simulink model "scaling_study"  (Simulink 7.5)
settings: Solver=ode23t  StartTime=0.0  StopTime=6  RelTol=1e-6
undefined symbols (not defined in the file or in its folder): dfilt, DiscIntNeverNeededParam
libraries: powerlib x45, powerlib_extras x17, simulink x12, dsparch4 x2
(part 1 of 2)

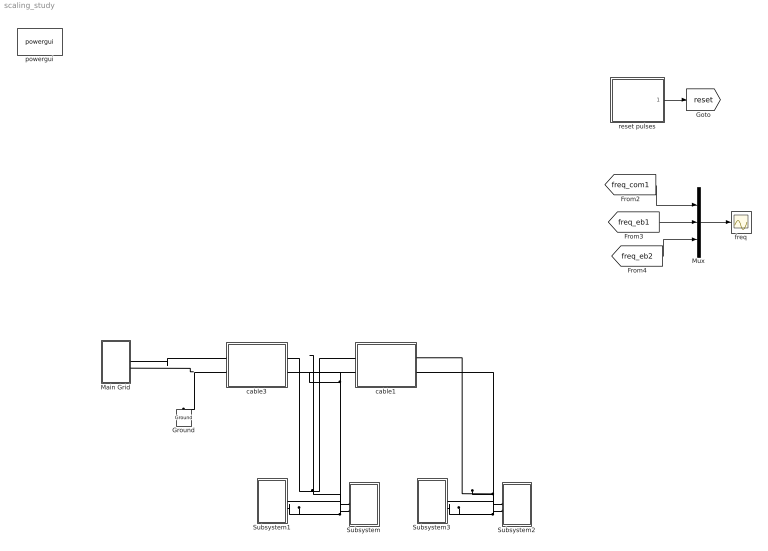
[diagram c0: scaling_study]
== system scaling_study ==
  Ground : powerlib/Elements/Ground  DialogController=POWERSYS.PowerSysDialog  PhysicalDomain=powersysdomain  SubClassName=unknown  LeftPortType=p1  RightPortType=p1  LConnTagsString=a
  Main Grid : Subsystem
  Mux : Mux  Inputs=3
  Subsystem : Subsystem
  Subsystem1 : Subsystem
  Subsystem2 : Subsystem
  Subsystem3 : Subsystem
  cable1 : Subsystem
  cable3 : Subsystem
  freq : Scope
  powergui : powerlib/powergui  Priority=1  SystemSampleTime=-1  SimulationMode=Discrete  SampleTime=50e-5  frequency=60  SPID=off  DisableSnubberDevices=off  DisableRonSwitches=off  DisableVfSwitches=off  SwTol=0  Interpol=off  frequencyindice=0  echomessages=off  HookPort=off  DisplayEquations=off  FunctionMessages=off  EnableUseOfTLC=off  x0status=blocks  RestoreLinks=warning  ResistiveCurrentMeasurement=off  Frange=[0:2:500]  Ylog=off  Xlog=on  ShowGrid=off  save=off  variable=ZData  ZoomFFT=on  StartTime=0.0  cycles=1  DisplayStyle=1  fundamental=60  FreqAxis=off  MaxFrequency=1000  frequencyindicesteady=1  RmsSteady=1  display=off  Ts=0  methode=off
  reset pulses : Subsystem  mask{tpulse=[50 100]}
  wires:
  Mux/1 -> freq/1
  reset pulses/1(Out1) -> [reset]
  [freq_com1] -> Mux/1
  [freq_eb1] -> Mux/2
  [freq_eb2] -> Mux/3
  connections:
  Main Grid/LConn1 -- cable3/RConn1
  cable3/RConn2 -- Main Grid/LConn2 -- Ground/LConn1
  Subsystem/LConn1 -- cable3/LConn1 -- cable1/RConn1 -- Subsystem1/LConn1
  Subsystem/LConn2 -- cable3/LConn2 -- cable1/RConn2 -- Subsystem1/LConn2
  Subsystem2/LConn1 -- cable1/LConn1 -- Subsystem3/LConn1
  Subsystem2/LConn2 -- cable1/LConn2 -- Subsystem3/LConn2

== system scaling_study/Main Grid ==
  " main-grid" : Scope  NumInputPorts=4
  Breaker : powerlib/Elements/Breaker  DialogController=POWERSYS.PowerSysDialog  SystemSampleTime=-1  BreakerResistance=0.01  InitialState=1  SnubberResistance=1e6  SnubberCapacitance=inf  SwitchingTimes=[5]  External=off  Measurements=None  MoreParameters=off  NoBreakLoop=off
  Main Grid 240V rms : powerlib/Electrical Sources/AC Voltage Source  DialogController=POWERSYS.PowerSysDialog  SystemSampleTime=-1  Amplitude=240*sqrt(2)  Phase=0  Frequency=60  SampleTime=0  Measurements=None
  cable : Subsystem
  measurement feeder C5 : Subsystem
  Conn1 : PMIOPort  Port=1  Side=Left
  Conn2 : PMIOPort  Port=2  Side=Left
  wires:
  measurement feeder C5/1(Vm) -> " main-grid"/1
  measurement feeder C5/2(Im) -> " main-grid"/2
  measurement feeder C5/3(PQ) -> " main-grid"/3
  measurement feeder C5/4(RMS (V-I)) -> " main-grid"/4
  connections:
  measurement feeder C5/RConn1 -- Breaker/LConn1
  cable/RConn1 -- Breaker/RConn1
  measurement feeder C5/LConn2 -- Main Grid 240V rms/LConn1
  measurement feeder C5/LConn1 -- Main Grid 240V rms/RConn1
  cable/RConn2 -- measurement feeder C5/RConn2
  Conn1/RConn1 -- cable/LConn1
  Conn2/RConn1 -- cable/LConn2

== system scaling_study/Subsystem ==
  120 Watt  e-board3 : Subsystem  mask{tf=100, p=1}
      mask prompts: tf "fault_time"; p "load priority"
  Breaker2 : powerlib/Elements/Breaker  DialogController=POWERSYS.PowerSysDialog  SystemSampleTime=-1  BreakerResistance=0.01  InitialState=1  SnubberResistance=1e6  SnubberCapacitance=inf  SwitchingTimes=[100]  External=off  Measurements=None  MoreParameters=off  NoBreakLoop=off
  eboard3 : Scope  NumInputPorts=4
  A : PMIOPort  Port=1  Side=Left
  C : PMIOPort  Port=2  Side=Left
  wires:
  120 Watt  e-board3/1(w) -> eboard3/1
  120 Watt  e-board3/2(Irms) -> eboard3/2
  120 Watt  e-board3/3(Vrms) -> eboard3/3
  [reset] -> 120 Watt  e-board3/1(reset)
  120 Watt  e-board3/4(Pload) -> eboard3/4, [Pload3]
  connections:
  120 Watt  e-board3/LConn1 -- Breaker2/LConn1
  A/RConn1 -- Breaker2/RConn1
  C/RConn1 -- 120 Watt  e-board3/LConn2

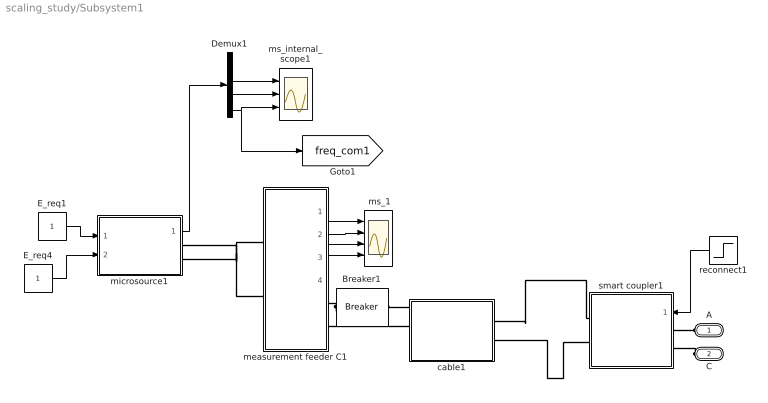
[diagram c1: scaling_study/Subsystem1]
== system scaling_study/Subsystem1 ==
  " ms_1" : Scope  NumInputPorts=4
  Breaker1 : powerlib/Elements/Breaker  DialogController=POWERSYS.PowerSysDialog  SystemSampleTime=-1  BreakerResistance=0.01  InitialState=1  SnubberResistance=1e6  SnubberCapacitance=inf  SwitchingTimes=[100]  External=off  Measurements=None  MoreParameters=off  NoBreakLoop=off
  Demux1 : Demux  Outputs=3
  E_req1 : Constant  OutDataType=fixdt(1, 16)  OutScaling=2^0
  E_req4 : Constant  OutDataType=fixdt(1, 16)  OutScaling=2^0
  cable1 : Subsystem
  measurement feeder C1 : Subsystem
  microsource1 : Subsystem  AncestorBlock=|
      | UWM_blocks/inverter-based
      | DG (simplified)
      | 208V - 15kVA
  ms_internal_scope1 : Scope  NumInputPorts=3
  reconnect1 : Step  Time=.1  SampleTime=0
  smart coupler1 : Subsystem
  A : PMIOPort  Port=1  Side=Left
  C : PMIOPort  Port=2  Side=Left
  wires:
  measurement feeder C1/1(Vm) -> " ms_1"/1
  measurement feeder C1/2(Im) -> " ms_1"/2
  measurement feeder C1/3(PQ) -> " ms_1"/3
  measurement feeder C1/4(RMS (V-I)) -> " ms_1"/4
  E_req1/1 -> microsource1/1(E_req)
  Demux1/2 -> ms_internal_scope1/2
  Demux1/1 -> ms_internal_scope1/1
  Demux1/3 -> ms_internal_scope1/3, [freq_com1]
  microsource1/1(m) -> Demux1/1
  reconnect1/1 -> smart coupler1/1(switch)
  E_req4/1 -> microsource1/2(P_req)
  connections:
  cable1/RConn1 -- Breaker1/LConn1
  Breaker1/RConn1 -- measurement feeder C1/RConn1
  smart coupler1/RConn1 -- cable1/LConn1
  cable1/LConn2 -- smart coupler1/RConn2
  cable1/RConn2 -- measurement feeder C1/RConn2
  measurement feeder C1/LConn1 -- microsource1/RConn1
  measurement feeder C1/LConn2 -- microsource1/RConn2
  A/RConn1 -- smart coupler1/LConn1
  C/RConn1 -- smart coupler1/LConn2

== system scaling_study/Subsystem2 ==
  120 Watt  e-board3 : Subsystem  mask{tf=100, p=1}
      mask prompts: tf "fault_time"; p "load priority"
  Breaker2 : powerlib/Elements/Breaker  DialogController=POWERSYS.PowerSysDialog  SystemSampleTime=-1  BreakerResistance=0.01  InitialState=1  SnubberResistance=1e6  SnubberCapacitance=inf  SwitchingTimes=[100]  External=off  Measurements=None  MoreParameters=off  NoBreakLoop=off
  eboard3 : Scope  NumInputPorts=4
  A : PMIOPort  Port=1  Side=Left
  C : PMIOPort  Port=2  Side=Left
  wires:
  120 Watt  e-board3/1(w) -> eboard3/1
  120 Watt  e-board3/2(Irms) -> eboard3/2
  120 Watt  e-board3/3(Vrms) -> eboard3/3
  [reset] -> 120 Watt  e-board3/1(reset)
  120 Watt  e-board3/4(Pload) -> eboard3/4, [Pload3]
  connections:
  120 Watt  e-board3/LConn1 -- Breaker2/LConn1
  A/RConn1 -- Breaker2/RConn1
  C/RConn1 -- 120 Watt  e-board3/LConn2

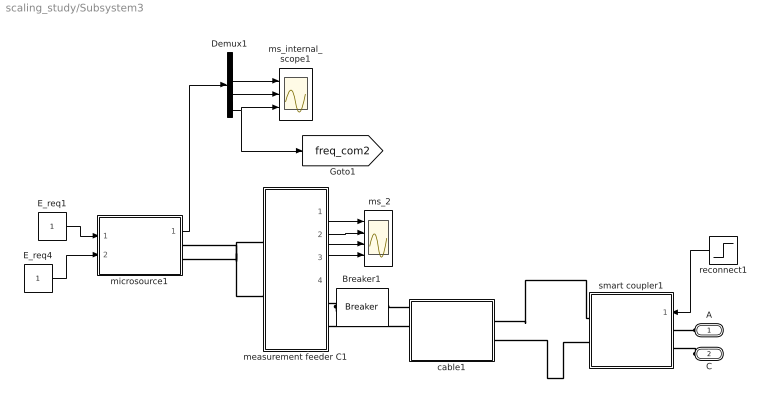
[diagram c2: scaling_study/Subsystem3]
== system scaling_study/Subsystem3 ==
  " ms_2" : Scope  NumInputPorts=4
  Breaker1 : powerlib/Elements/Breaker  DialogController=POWERSYS.PowerSysDialog  SystemSampleTime=-1  BreakerResistance=0.01  InitialState=1  SnubberResistance=1e6  SnubberCapacitance=inf  SwitchingTimes=[100]  External=off  Measurements=None  MoreParameters=off  NoBreakLoop=off
  Demux1 : Demux  Outputs=3
  E_req1 : Constant  OutDataType=fixdt(1, 16)  OutScaling=2^0
  E_req4 : Constant  OutDataType=fixdt(1, 16)  OutScaling=2^0
  cable1 : Subsystem
  measurement feeder C1 : Subsystem
  microsource1 : Subsystem  AncestorBlock=|
      | UWM_blocks/inverter-based
      | DG (simplified)
      | 208V - 15kVA
  ms_internal_scope1 : Scope  NumInputPorts=3
  reconnect1 : Step  Time=.1  SampleTime=0
  smart coupler1 : Subsystem
  A : PMIOPort  Port=1  Side=Left
  C : PMIOPort  Port=2  Side=Left
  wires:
  measurement feeder C1/1(Vm) -> " ms_2"/1
  measurement feeder C1/2(Im) -> " ms_2"/2
  measurement feeder C1/3(PQ) -> " ms_2"/3
  measurement feeder C1/4(RMS (V-I)) -> " ms_2"/4
  E_req1/1 -> microsource1/1(E_req)
  Demux1/2 -> ms_internal_scope1/2
  Demux1/1 -> ms_internal_scope1/1
  Demux1/3 -> ms_internal_scope1/3, [freq_com2]
  microsource1/1(m) -> Demux1/1
  reconnect1/1 -> smart coupler1/1(switch)
  E_req4/1 -> microsource1/2(P_req)
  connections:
  cable1/RConn1 -- Breaker1/LConn1
  Breaker1/RConn1 -- measurement feeder C1/RConn1
  smart coupler1/RConn1 -- cable1/LConn1
  cable1/LConn2 -- smart coupler1/RConn2
  cable1/RConn2 -- measurement feeder C1/RConn2
  measurement feeder C1/LConn1 -- microsource1/RConn1
  measurement feeder C1/LConn2 -- microsource1/RConn2
  A/RConn1 -- smart coupler1/LConn1
  C/RConn1 -- smart coupler1/LConn2

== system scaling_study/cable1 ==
  Series RLC Branch : powerlib/Elements/Series RLC Branch  DialogController=POWERSYS.PowerSysDialog  PhysicalDomain=powersysdomain  SubClassName=unknown  LeftPortType=p1  RightPortType=p1  LConnTagsString=__new0  RConnTagsString=__new0  BranchType=RL  Resistance=.001  Inductance=1.e-6  SetiL0=off  InitialCurrent=0  Capacitance=1e-6  Setx0=off  InitialVoltage=0  Measurements=None
  A : PMIOPort  Tag=PMCPort  Port=1  Side=Left
  A' : PMIOPort  Tag=PMCPort  Port=2  Side=Right
  B' : PMIOPort  Tag=PMCPort  Port=3  Side=Right
  B : PMIOPort  Tag=PMCPort  Port=4  Side=Left
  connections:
  A/RConn1 -- Series RLC Branch/LConn1
  Series RLC Branch/RConn1 -- A'/RConn1
  B/RConn1 -- B'/RConn1

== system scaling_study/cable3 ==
  Series RLC Branch : powerlib/Elements/Series RLC Branch  DialogController=POWERSYS.PowerSysDialog  PhysicalDomain=powersysdomain  SubClassName=unknown  LeftPortType=p1  RightPortType=p1  LConnTagsString=__new0  RConnTagsString=__new0  BranchType=RL  Resistance=.001  Inductance=1.e-6  SetiL0=off  InitialCurrent=0  Capacitance=1e-6  Setx0=off  InitialVoltage=0  Measurements=None
  A : PMIOPort  Tag=PMCPort  Port=1  Side=Left
  A' : PMIOPort  Tag=PMCPort  Port=2  Side=Right
  B' : PMIOPort  Tag=PMCPort  Port=3  Side=Right
  B : PMIOPort  Tag=PMCPort  Port=4  Side=Left
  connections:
  A/RConn1 -- Series RLC Branch/LConn1
  Series RLC Branch/RConn1 -- A'/RConn1
  B/RConn1 -- B'/RConn1

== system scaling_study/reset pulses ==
  Sum : Sum  Inputs=|++  OutDataType=fixdt(1, 16)  OutScaling=2^0
  pulse : Subsystem  mask{tstart=tpulse(1), dt=.1}
  pulse1 : Subsystem  mask{tstart=tpulse(2), dt=.1}
  Out1 : Outport
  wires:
  pulse/1(Out1) -> Sum/1
  pulse1/1(Out1) -> Sum/2
  Sum/1 -> Out1/1

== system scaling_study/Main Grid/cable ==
  Series RLC Branch : powerlib/Elements/Series RLC Branch  DialogController=POWERSYS.PowerSysDialog  PhysicalDomain=powersysdomain  SubClassName=unknown  LeftPortType=p1  RightPortType=p1  LConnTagsString=__new0  RConnTagsString=__new0  BranchType=RL  Resistance=.001  Inductance=1.e-5  SetiL0=off  InitialCurrent=0  Capacitance=1e-6  Setx0=off  InitialVoltage=0  Measurements=None
  A : PMIOPort  Tag=PMCPort  Port=1  Side=Left
  A' : PMIOPort  Tag=PMCPort  Port=2  Side=Right
  B' : PMIOPort  Tag=PMCPort  Port=3  Side=Right
  B : PMIOPort  Tag=PMCPort  Port=4  Side=Left
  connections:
  A/RConn1 -- Series RLC Branch/LConn1
  A'/RConn1 -- Series RLC Branch/RConn1
  B/RConn1 -- B'/RConn1

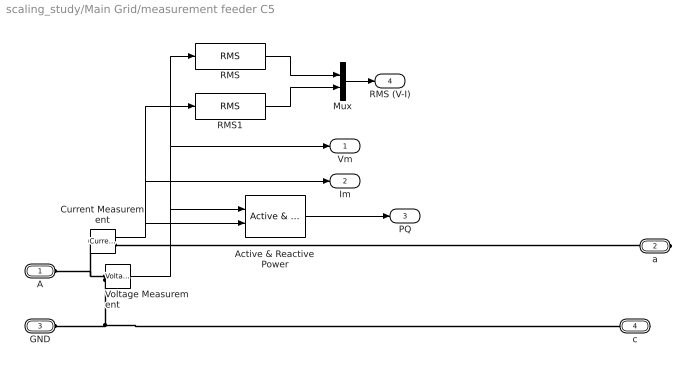
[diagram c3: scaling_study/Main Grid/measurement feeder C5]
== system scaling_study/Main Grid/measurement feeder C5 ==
  Active & Reactive Power : powerlib_extras/Measurements/Active & Reactive Power  DialogController=POWERSYS.PowerSysDialog  SystemSampleTime=-1  f1=60
  Current Measurement : powerlib/Measurements/Current Measurement  DialogController=POWERSYS.PowerSysDialog  SystemSampleTime=-1  PhasorSimulation=off  OutputType=Complex  PSBequivalent=0
  Mux : Mux  Inputs=2
  RMS : powerlib_extras/Measurements/RMS  DialogController=POWERSYS.PowerSysDialog  SystemSampleTime=-1  f1=60
  RMS1 : powerlib_extras/Measurements/RMS  DialogController=POWERSYS.PowerSysDialog  SystemSampleTime=-1  f1=60
  Voltage Measurement : powerlib/Measurements/Voltage Measurement  DialogController=POWERSYS.PowerSysDialog  SystemSampleTime=-1  PhasorSimulation=off  OutputType=Complex  PSBequivalent=0
  A : PMIOPort  Port=1  Side=Left
  a : PMIOPort  Port=2  Side=Right
  GND : PMIOPort  Port=3  Side=Left
  c : PMIOPort  Port=4  Side=Right
  Vm : Outport  OutDataType=fixdt(1, 16)  OutScaling=2^0
  Im : Outport  Port=2  OutDataType=fixdt(1, 16)  OutScaling=2^0
  PQ : Outport  Port=3  OutDataType=fixdt(1, 16)  OutScaling=2^0
  RMS (V-I) : Outport  Port=4  OutDataType=fixdt(1, 16)  OutScaling=2^0
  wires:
  Mux/1 -> RMS (V-I)/1
  Current Measurement/1 -> Im/1, RMS1/1, Active & Reactive Power/2
  Voltage Measurement/1 -> Vm/1, RMS/1, Active & Reactive Power/1
  Active & Reactive Power/1 -> PQ/1
  RMS/1 -> Mux/1
  RMS1/1 -> Mux/2
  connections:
  a/RConn1 -- Current Measurement/RConn1
  Voltage Measurement/LConn1 -- A/RConn1 -- Current Measurement/LConn1
  Voltage Measurement/LConn2 -- GND/RConn1 -- c/RConn1

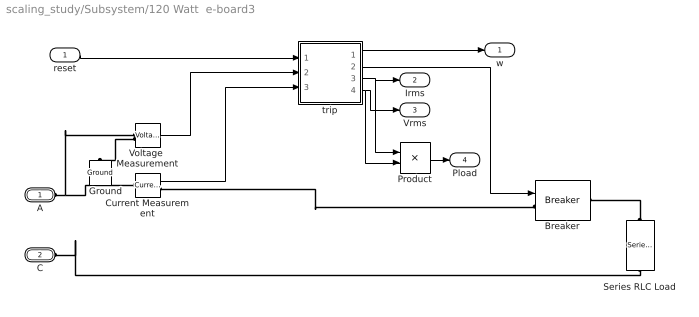
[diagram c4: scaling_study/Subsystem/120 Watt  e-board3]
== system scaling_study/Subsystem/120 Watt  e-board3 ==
  reset : Inport
  Breaker : powerlib/Elements/Breaker  DialogController=POWERSYS.PowerSysDialog  SystemSampleTime=-1  BreakerResistance=0.01  InitialState=1  SnubberResistance=1e6  SnubberCapacitance=inf  SwitchingTimes="[ 1/60  5/60 ]"  External=on  Measurements=None  MoreParameters=off  NoBreakLoop=off
  Current Measurement : powerlib/Measurements/Current Measurement  DialogController=POWERSYS.PowerSysDialog  SystemSampleTime=-1  PhasorSimulation=off  OutputType=Complex  PSBequivalent=0
  Ground : powerlib/Elements/Ground  DialogController=POWERSYS.PowerSysDialog  PhysicalDomain=powersysdomain  SubClassName=unknown  LeftPortType=p1  RightPortType=p1  LConnTagsString=a
  Product : Product  OutDataType=fixdt(1, 16)  OutScaling=2^0
  Series RLC Load : powerlib/Elements/Series RLC Load  DialogController=POWERSYS.PowerSysDialog  PhysicalDomain=powersysdomain  SubClassName=unknown  LeftPortType=p1  RightPortType=p1  LConnTagsString=a  RConnTagsString=__new0  NominalVoltage=240  NominalFrequency=60  ActivePower=120  InductivePower=0  CapacitivePower=0  Setx0=off  InitialVoltage=0  SetiL0=off  InitialCurrent=0  Measurements=None
  Voltage  Measurement : powerlib/Measurements/Voltage Measurement  DialogController=POWERSYS.PowerSysDialog  SystemSampleTime=-1  PhasorSimulation=off  OutputType=Complex  PSBequivalent=0
  trip : Subsystem  mask{p=p}
      mask prompts: p "priority level"
  A : PMIOPort  Port=1  Side=Left
  C : PMIOPort  Port=2  Side=Left
  w : Outport  OutDataType=fixdt(1, 16)  OutScaling=2^0
  Irms : Outport  Port=2  OutDataType=fixdt(1, 16)  OutScaling=2^0
  Vrms : Outport  Port=3  OutDataType=fixdt(1, 16)  OutScaling=2^0
  Pload : Outport  Port=4  OutDataType=fixdt(1, 16)  OutScaling=2^0
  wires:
  trip/1(w) -> w/1
  Current Measurement/1 -> trip/3(I)
  Voltage  Measurement/1 -> trip/2(V)
  reset/1 -> trip/1(Reset)
  trip/2(trip) -> Breaker/1
  trip/3(Irms) -> Irms/1, Product/1
  trip/4(Vrms) -> Vrms/1, Product/2
  Product/1 -> Pload/1
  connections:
  A/RConn1 -- Current Measurement/LConn1 -- Voltage  Measurement/LConn1
  Voltage  Measurement/LConn2 -- Ground/LConn1
  Current Measurement/RConn1 -- Breaker/LConn1
  Series RLC Load/LConn1 -- Breaker/RConn1
  Series RLC Load/RConn1 -- C/RConn1

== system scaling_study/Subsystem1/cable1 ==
  Series RLC Branch : powerlib/Elements/Series RLC Branch  DialogController=POWERSYS.PowerSysDialog  PhysicalDomain=powersysdomain  SubClassName=unknown  LeftPortType=p1  RightPortType=p1  LConnTagsString=__new0  RConnTagsString=__new0  BranchType=RL  Resistance=.001  Inductance=1.e-6  SetiL0=off  InitialCurrent=0  Capacitance=1e-6  Setx0=off  InitialVoltage=0  Measurements=None
  A : PMIOPort  Tag=PMCPort  Port=1  Side=Left
  A' : PMIOPort  Tag=PMCPort  Port=2  Side=Right
  B' : PMIOPort  Tag=PMCPort  Port=3  Side=Right
  B : PMIOPort  Tag=PMCPort  Port=4  Side=Left
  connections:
  A/RConn1 -- Series RLC Branch/LConn1
  Series RLC Branch/RConn1 -- A'/RConn1
  B/RConn1 -- B'/RConn1

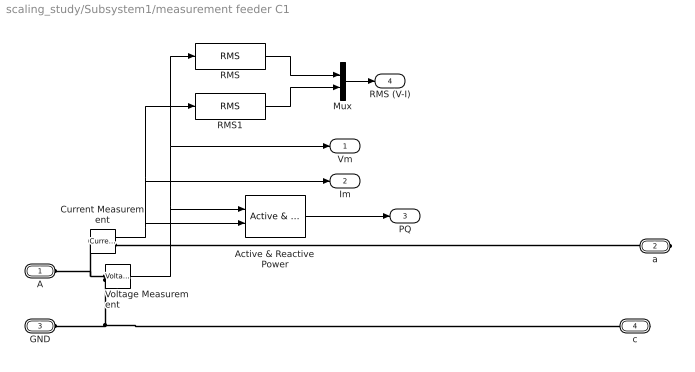
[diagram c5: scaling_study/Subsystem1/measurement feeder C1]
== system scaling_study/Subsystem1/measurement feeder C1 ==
  Active & Reactive Power : powerlib_extras/Measurements/Active & Reactive Power  DialogController=POWERSYS.PowerSysDialog  SystemSampleTime=-1  f1=60
  Current Measurement : powerlib/Measurements/Current Measurement  DialogController=POWERSYS.PowerSysDialog  SystemSampleTime=-1  PhasorSimulation=off  OutputType=Complex  PSBequivalent=0
  Mux : Mux  Inputs=2
  RMS : powerlib_extras/Measurements/RMS  DialogController=POWERSYS.PowerSysDialog  SystemSampleTime=-1  f1=60
  RMS1 : powerlib_extras/Measurements/RMS  DialogController=POWERSYS.PowerSysDialog  SystemSampleTime=-1  f1=60
  Voltage Measurement : powerlib/Measurements/Voltage Measurement  DialogController=POWERSYS.PowerSysDialog  SystemSampleTime=-1  PhasorSimulation=off  OutputType=Complex  PSBequivalent=0
  A : PMIOPort  Port=1  Side=Left
  a : PMIOPort  Port=2  Side=Right
  GND : PMIOPort  Port=3  Side=Left
  c : PMIOPort  Port=4  Side=Right
  Vm : Outport  OutDataType=fixdt(1, 16)  OutScaling=2^0
  Im : Outport  Port=2  OutDataType=fixdt(1, 16)  OutScaling=2^0
  PQ : Outport  Port=3  OutDataType=fixdt(1, 16)  OutScaling=2^0
  RMS (V-I) : Outport  Port=4  OutDataType=fixdt(1, 16)  OutScaling=2^0
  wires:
  Mux/1 -> RMS (V-I)/1
  Current Measurement/1 -> Im/1, RMS1/1, Active & Reactive Power/2
  Voltage Measurement/1 -> Vm/1, RMS/1, Active & Reactive Power/1
  Active & Reactive Power/1 -> PQ/1
  RMS/1 -> Mux/1
  RMS1/1 -> Mux/2
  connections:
  a/RConn1 -- Current Measurement/RConn1
  Voltage Measurement/LConn1 -- A/RConn1 -- Current Measurement/LConn1
  Voltage Measurement/LConn2 -- GND/RConn1 -- c/RConn1

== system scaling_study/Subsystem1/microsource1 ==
  E_req : Inport
  P_req : Inport  Port=2
  Current Measurement : powerlib/Measurements/Current Measurement  DialogController=POWERSYS.PowerSysDialog  SystemSampleTime=-1  PhasorSimulation=off  OutputType=Complex  PSBequivalent=0
  Gain : Gain  Gain=1/(2*pi)  ParameterDataType=fixdt(1, 16)  ParameterScaling=2^0  OutDataType=fixdt(1, 16)  OutScaling=2^0
  Mux : Mux  Inputs=3
  Parallel RLC Branch : powerlib/Elements/Parallel RLC Branch  DialogController=POWERSYS.PowerSysDialog  PhysicalDomain=powersysdomain  SubClassName=unknown  LeftPortType=p1  RightPortType=p1  LConnTagsString=a  RConnTagsString=__new0  BranchType=L  Resistance=1  Inductance=1.e-1  SetiL0=off  InitialCurrent=0  Capacitance=1e-6  Setx0=off  InitialVoltage=0  Measurements=None
  Parallel RLC Branch1 : powerlib/Elements/Parallel RLC Branch  DialogController=POWERSYS.PowerSysDialog  PhysicalDomain=powersysdomain  SubClassName=unknown  LeftPortType=p1  RightPortType=p1  LConnTagsString=a  RConnTagsString=__new0  BranchType=L  Resistance=1  Inductance=1.e-1  SetiL0=off  InitialCurrent=0  Capacitance=1e-6  Setx0=off  InitialVoltage=0  Measurements=None
  Parallel RLC Branch2 : powerlib/Elements/Parallel RLC Branch  DialogController=POWERSYS.PowerSysDialog  PhysicalDomain=powersysdomain  SubClassName=unknown  LeftPortType=p1  RightPortType=p1  LConnTagsString=a  RConnTagsString=__new0  BranchType=C  Resistance=1  Inductance=1.e-1  SetiL0=off  InitialCurrent=0  Capacitance=1.e-5  Setx0=off  InitialVoltage=0  Measurements=None
  UWM_controller : Subsystem  mask{Vbase=240*sqrt(2), Sbase=200}
  Voltage Measurement : powerlib/Measurements/Voltage Measurement  DialogController=POWERSYS.PowerSysDialog  SystemSampleTime=-1  PhasorSimulation=off  OutputType=Complex  PSBequivalent=0
  microsource : Subsystem
  a : PMIOPort  Port=1  Side=Right
  GND : PMIOPort  Port=2  Side=Right
  m : Outport  OutDataType=fixdt(1, 16)  OutScaling=2^0
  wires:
  E_req/1 -> UWM_controller/3(E_req)
  P_req/1 -> UWM_controller/4(P_req)
  UWM_controller/1(Vpk) -> microsource/1(Vpk)
  UWM_controller/2(w) -> microsource/2(w), Gain/1
  Mux/1 -> m/1
  Gain/1 -> Mux/3
  Current Measurement/1 -> Mux/2, UWM_controller/2(i_meas)
  Voltage Measurement/1 -> Mux/1, UWM_controller/1(v_meas)
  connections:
  Voltage Measurement/LConn2 -- GND/RConn1 -- Parallel RLC Branch2/RConn1 -- microsource/RConn2
  Parallel RLC Branch1/RConn1 -- Voltage Measurement/LConn1 -- Current Measurement/LConn1
  a/RConn1 -- Current Measurement/RConn1
  Parallel RLC Branch/LConn1 -- microsource/RConn1
  Parallel RLC Branch2/LConn1 -- Parallel RLC Branch1/LConn1 -- Parallel RLC Branch/RConn1

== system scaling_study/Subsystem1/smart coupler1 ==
  switch : Inport  OutDataType=fixdt(1, 16)  OutScaling=2^0
  Abs : Abs  OutDataType=fixdt(1, 16)  OutScaling=2^0
  Breaker : powerlib/Elements/Breaker  DialogController=POWERSYS.PowerSysDialog  SystemSampleTime=-1  BreakerResistance=0.01  InitialState=0  SnubberResistance=1e6  SnubberCapacitance=inf  SwitchingTimes="[ 1/60  5/60 ]"  External=on  Measurements=None  MoreParameters=off  NoBreakLoop=off
  Level-2 M-file S-Function : M-S-Function  FunctionName=smart_coupler
  Scope : Scope  NumInputPorts=3
  Transfer Fcn : TransferFcn  Numerator=[100]  Denominator=[1 100]
  Voltage Measurement : powerlib/Measurements/Voltage Measurement  DialogController=POWERSYS.PowerSysDialog  SystemSampleTime=-1  PhasorSimulation=off  OutputType=Complex  PSBequivalent=0
  A : PMIOPort  Port=1  Side=Left
  C : PMIOPort  Port=2  Side=Left
  a : PMIOPort  Port=3  Side=Right
  c : PMIOPort  Port=4  Side=Right
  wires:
  switch/1 -> Level-2 M-file S-Function/2, Scope/2
  Level-2 M-file S-Function/1 -> Scope/1, Breaker/1
  Voltage Measurement/1 -> Abs/1
  Abs/1 -> Transfer Fcn/1
  Transfer Fcn/1 -> Level-2 M-file S-Function/1, Scope/3
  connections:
  Breaker/LConn1 -- A/RConn1 -- Voltage Measurement/LConn1
  Breaker/RConn1 -- Voltage Measurement/LConn2 -- a/RConn1
  c/RConn1 -- C/RConn1

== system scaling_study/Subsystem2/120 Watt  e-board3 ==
  reset : Inport
  Breaker : powerlib/Elements/Breaker  DialogController=POWERSYS.PowerSysDialog  SystemSampleTime=-1  BreakerResistance=0.01  InitialState=1  SnubberResistance=1e6  SnubberCapacitance=inf  SwitchingTimes="[ 1/60  5/60 ]"  External=on  Measurements=None  MoreParameters=off  NoBreakLoop=off
  Current Measurement : powerlib/Measurements/Current Measurement  DialogController=POWERSYS.PowerSysDialog  SystemSampleTime=-1  PhasorSimulation=off  OutputType=Complex  PSBequivalent=0
  Ground : powerlib/Elements/Ground  DialogController=POWERSYS.PowerSysDialog  PhysicalDomain=powersysdomain  SubClassName=unknown  LeftPortType=p1  RightPortType=p1  LConnTagsString=a
  Product : Product  OutDataType=fixdt(1, 16)  OutScaling=2^0
  Series RLC Load : powerlib/Elements/Series RLC Load  DialogController=POWERSYS.PowerSysDialog  PhysicalDomain=powersysdomain  SubClassName=unknown  LeftPortType=p1  RightPortType=p1  LConnTagsString=a  RConnTagsString=__new0  NominalVoltage=240  NominalFrequency=60  ActivePower=120  InductivePower=0  CapacitivePower=0  Setx0=off  InitialVoltage=0  SetiL0=off  InitialCurrent=0  Measurements=None
  Voltage  Measurement : powerlib/Measurements/Voltage Measurement  DialogController=POWERSYS.PowerSysDialog  SystemSampleTime=-1  PhasorSimulation=off  OutputType=Complex  PSBequivalent=0
  trip : Subsystem  mask{p=p}
      mask prompts: p "priority level"
  A : PMIOPort  Port=1  Side=Left
  C : PMIOPort  Port=2  Side=Left
  w : Outport  OutDataType=fixdt(1, 16)  OutScaling=2^0
  Irms : Outport  Port=2  OutDataType=fixdt(1, 16)  OutScaling=2^0
  Vrms : Outport  Port=3  OutDataType=fixdt(1, 16)  OutScaling=2^0
  Pload : Outport  Port=4  OutDataType=fixdt(1, 16)  OutScaling=2^0
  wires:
  trip/1(w) -> w/1
  Current Measurement/1 -> trip/3(I)
  Voltage  Measurement/1 -> trip/2(V)
  reset/1 -> trip/1(Reset)
  trip/2(trip) -> Breaker/1
  trip/3(Irms) -> Irms/1, Product/1
  trip/4(Vrms) -> Vrms/1, Product/2
  Product/1 -> Pload/1
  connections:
  A/RConn1 -- Current Measurement/LConn1 -- Voltage  Measurement/LConn1
  Voltage  Measurement/LConn2 -- Ground/LConn1
  Current Measurement/RConn1 -- Breaker/LConn1
  Series RLC Load/LConn1 -- Breaker/RConn1
  Series RLC Load/RConn1 -- C/RConn1

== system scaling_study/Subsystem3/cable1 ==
  Series RLC Branch : powerlib/Elements/Series RLC Branch  DialogController=POWERSYS.PowerSysDialog  PhysicalDomain=powersysdomain  SubClassName=unknown  LeftPortType=p1  RightPortType=p1  LConnTagsString=__new0  RConnTagsString=__new0  BranchType=RL  Resistance=.001  Inductance=1.e-6  SetiL0=off  InitialCurrent=0  Capacitance=1e-6  Setx0=off  InitialVoltage=0  Measurements=None
  A : PMIOPort  Tag=PMCPort  Port=1  Side=Left
  A' : PMIOPort  Tag=PMCPort  Port=2  Side=Right
  B' : PMIOPort  Tag=PMCPort  Port=3  Side=Right
  B : PMIOPort  Tag=PMCPort  Port=4  Side=Left
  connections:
  A/RConn1 -- Series RLC Branch/LConn1
  Series RLC Branch/RConn1 -- A'/RConn1
  B/RConn1 -- B'/RConn1

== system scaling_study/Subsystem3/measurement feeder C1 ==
  Active & Reactive Power : powerlib_extras/Measurements/Active & Reactive Power  DialogController=POWERSYS.PowerSysDialog  SystemSampleTime=-1  f1=60
  Current Measurement : powerlib/Measurements/Current Measurement  DialogController=POWERSYS.PowerSysDialog  SystemSampleTime=-1  PhasorSimulation=off  OutputType=Complex  PSBequivalent=0
  Mux : Mux  Inputs=2
  RMS : powerlib_extras/Measurements/RMS  DialogController=POWERSYS.PowerSysDialog  SystemSampleTime=-1  f1=60
  RMS1 : powerlib_extras/Measurements/RMS  DialogController=POWERSYS.PowerSysDialog  SystemSampleTime=-1  f1=60
  Voltage Measurement : powerlib/Measurements/Voltage Measurement  DialogController=POWERSYS.PowerSysDialog  SystemSampleTime=-1  PhasorSimulation=off  OutputType=Complex  PSBequivalent=0
  A : PMIOPort  Port=1  Side=Left
  a : PMIOPort  Port=2  Side=Right
  GND : PMIOPort  Port=3  Side=Left
  c : PMIOPort  Port=4  Side=Right
  Vm : Outport  OutDataType=fixdt(1, 16)  OutScaling=2^0
  Im : Outport  Port=2  OutDataType=fixdt(1, 16)  OutScaling=2^0
  PQ : Outport  Port=3  OutDataType=fixdt(1, 16)  OutScaling=2^0
  RMS (V-I) : Outport  Port=4  OutDataType=fixdt(1, 16)  OutScaling=2^0
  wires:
  Mux/1 -> RMS (V-I)/1
  Current Measurement/1 -> Im/1, RMS1/1, Active & Reactive Power/2
  Voltage Measurement/1 -> Vm/1, RMS/1, Active & Reactive Power/1
  Active & Reactive Power/1 -> PQ/1
  RMS/1 -> Mux/1
  RMS1/1 -> Mux/2
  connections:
  a/RConn1 -- Current Measurement/RConn1
  Voltage Measurement/LConn1 -- A/RConn1 -- Current Measurement/LConn1
  Voltage Measurement/LConn2 -- GND/RConn1 -- c/RConn1

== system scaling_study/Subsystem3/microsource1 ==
  E_req : Inport
  P_req : Inport  Port=2
  Current Measurement : powerlib/Measurements/Current Measurement  DialogController=POWERSYS.PowerSysDialog  SystemSampleTime=-1  PhasorSimulation=off  OutputType=Complex  PSBequivalent=0
  Gain : Gain  Gain=1/(2*pi)  ParameterDataType=fixdt(1, 16)  ParameterScaling=2^0  OutDataType=fixdt(1, 16)  OutScaling=2^0
  Mux : Mux  Inputs=3
  Parallel RLC Branch : powerlib/Elements/Parallel RLC Branch  DialogController=POWERSYS.PowerSysDialog  PhysicalDomain=powersysdomain  SubClassName=unknown  LeftPortType=p1  RightPortType=p1  LConnTagsString=a  RConnTagsString=__new0  BranchType=L  Resistance=1  Inductance=1.e-1  SetiL0=off  InitialCurrent=0  Capacitance=1e-6  Setx0=off  InitialVoltage=0  Measurements=None
  Parallel RLC Branch1 : powerlib/Elements/Parallel RLC Branch  DialogController=POWERSYS.PowerSysDialog  PhysicalDomain=powersysdomain  SubClassName=unknown  LeftPortType=p1  RightPortType=p1  LConnTagsString=a  RConnTagsString=__new0  BranchType=L  Resistance=1  Inductance=1.e-1  SetiL0=off  InitialCurrent=0  Capacitance=1e-6  Setx0=off  InitialVoltage=0  Measurements=None
  Parallel RLC Branch2 : powerlib/Elements/Parallel RLC Branch  DialogController=POWERSYS.PowerSysDialog  PhysicalDomain=powersysdomain  SubClassName=unknown  LeftPortType=p1  RightPortType=p1  LConnTagsString=a  RConnTagsString=__new0  BranchType=C  Resistance=1  Inductance=1.e-1  SetiL0=off  InitialCurrent=0  Capacitance=1.e-5  Setx0=off  InitialVoltage=0  Measurements=None
  UWM_controller : Subsystem  mask{Vbase=240*sqrt(2), Sbase=200}
  Voltage Measurement : powerlib/Measurements/Voltage Measurement  DialogController=POWERSYS.PowerSysDialog  SystemSampleTime=-1  PhasorSimulation=off  OutputType=Complex  PSBequivalent=0
  microsource : Subsystem
  a : PMIOPort  Port=1  Side=Right
  GND : PMIOPort  Port=2  Side=Right
  m : Outport  OutDataType=fixdt(1, 16)  OutScaling=2^0
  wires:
  E_req/1 -> UWM_controller/3(E_req)
  P_req/1 -> UWM_controller/4(P_req)
  UWM_controller/1(Vpk) -> microsource/1(Vpk)
  UWM_controller/2(w) -> microsource/2(w), Gain/1
  Mux/1 -> m/1
  Gain/1 -> Mux/3
  Current Measurement/1 -> Mux/2, UWM_controller/2(i_meas)
  Voltage Measurement/1 -> Mux/1, UWM_controller/1(v_meas)
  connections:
  Voltage Measurement/LConn2 -- GND/RConn1 -- Parallel RLC Branch2/RConn1 -- microsource/RConn2
  Parallel RLC Branch1/RConn1 -- Voltage Measurement/LConn1 -- Current Measurement/LConn1
  a/RConn1 -- Current Measurement/RConn1
  Parallel RLC Branch/LConn1 -- microsource/RConn1
  Parallel RLC Branch2/LConn1 -- Parallel RLC Branch1/LConn1 -- Parallel RLC Branch/RConn1

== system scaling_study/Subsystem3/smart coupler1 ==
  switch : Inport  OutDataType=fixdt(1, 16)  OutScaling=2^0
  Abs : Abs  OutDataType=fixdt(1, 16)  OutScaling=2^0
  Breaker : powerlib/Elements/Breaker  DialogController=POWERSYS.PowerSysDialog  SystemSampleTime=-1  BreakerResistance=0.01  InitialState=0  SnubberResistance=1e6  SnubberCapacitance=inf  SwitchingTimes="[ 1/60  5/60 ]"  External=on  Measurements=None  MoreParameters=off  NoBreakLoop=off
  Level-2 M-file S-Function : M-S-Function  FunctionName=smart_coupler
  Scope : Scope  NumInputPorts=3
  Transfer Fcn : TransferFcn  Numerator=[100]  Denominator=[1 100]
  Voltage Measurement : powerlib/Measurements/Voltage Measurement  DialogController=POWERSYS.PowerSysDialog  SystemSampleTime=-1  PhasorSimulation=off  OutputType=Complex  PSBequivalent=0
  A : PMIOPort  Port=1  Side=Left
  C : PMIOPort  Port=2  Side=Left
  a : PMIOPort  Port=3  Side=Right
  c : PMIOPort  Port=4  Side=Right
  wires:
  switch/1 -> Level-2 M-file S-Function/2, Scope/2
  Level-2 M-file S-Function/1 -> Scope/1, Breaker/1
  Voltage Measurement/1 -> Abs/1
  Abs/1 -> Transfer Fcn/1
  Transfer Fcn/1 -> Level-2 M-file S-Function/1, Scope/3
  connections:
  Breaker/LConn1 -- A/RConn1 -- Voltage Measurement/LConn1
  Breaker/RConn1 -- Voltage Measurement/LConn2 -- a/RConn1
  c/RConn1 -- C/RConn1

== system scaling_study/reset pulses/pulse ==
  Step : Step  Time=tstart  SampleTime=0
  Step1 : Step  Time=tstart+dt  After=-1  SampleTime=0
  Sum : Sum  Inputs=|++  OutDataType=fixdt(1, 16)  OutScaling=2^0
  Out1 : Outport
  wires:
  Step/1 -> Sum/2
  Step1/1 -> Sum/1
  Sum/1 -> Out1/1

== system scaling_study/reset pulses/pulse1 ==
  Step : Step  Time=tstart  SampleTime=0
  Step1 : Step  Time=tstart+dt  After=-1  SampleTime=0
  Sum : Sum  Inputs=|++  OutDataType=fixdt(1, 16)  OutScaling=2^0
  Out1 : Outport
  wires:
  Step/1 -> Sum/2
  Step1/1 -> Sum/1
  Sum/1 -> Out1/1

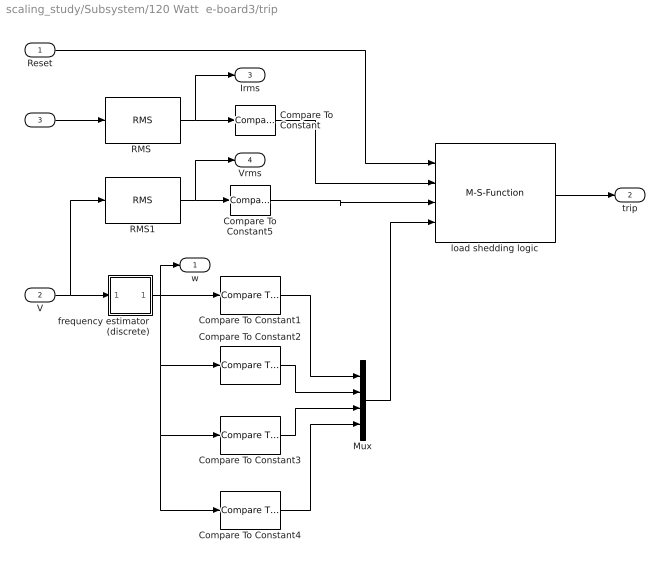
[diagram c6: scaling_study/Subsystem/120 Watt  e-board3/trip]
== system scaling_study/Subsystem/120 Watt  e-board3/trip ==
  Reset : Inport
  V : Inport  Port=2
  I : Inport  Port=3
  Compare To Constant : simulink/Logic and Bit Operations/Compare To Constant  SystemSampleTime=-1  relop=>=  const=100  LogicOutDataTypeMode=boolean
  Compare To Constant1 : simulink/Logic and Bit Operations/Compare To Constant  SystemSampleTime=-1  relop=<=  const=59.8  LogicOutDataTypeMode=boolean
  Compare To Constant2 : simulink/Logic and Bit Operations/Compare To Constant  SystemSampleTime=-1  relop=<=  const=59.5  LogicOutDataTypeMode=boolean
  Compare To Constant3 : simulink/Logic and Bit Operations/Compare To Constant  SystemSampleTime=-1  relop=>=  const=60.1  LogicOutDataTypeMode=boolean
  Compare To Constant4 : simulink/Logic and Bit Operations/Compare To Constant  SystemSampleTime=-1  relop=<=  const=58.6  LogicOutDataTypeMode=boolean
  Compare To Constant5 : simulink/Logic and Bit Operations/Compare To Constant  SystemSampleTime=-1  relop=<=  const=100  LogicOutDataTypeMode=boolean
  Mux : Mux
  "RMS " : powerlib_extras/Measurements/RMS  DialogController=POWERSYS.PowerSysDialog  SystemSampleTime=-1  f1=60
  RMS1 : powerlib_extras/Measurements/RMS  DialogController=POWERSYS.PowerSysDialog  SystemSampleTime=-1  f1=60
  frequency estimator (discrete) : Subsystem  mask{dt=0.010}
      mask prompts: dt "sample time"
  load shedding logic : M-S-Function  FunctionName=load_shedding_logic  Parameters=p
  w : Outport  OutDataType=fixdt(1, 16)  OutScaling=2^0
  trip : Outport  Port=2  DataType=double  OutDataTypeStr=double
  Irms : Outport  Port=3  OutDataType=fixdt(1, 16)  OutScaling=2^0
  Vrms : Outport  Port=4  OutDataType=fixdt(1, 16)  OutScaling=2^0
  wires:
  "RMS "/1 -> Compare To Constant/1, Irms/1
  I/1 -> "RMS "/1
  Reset/1 -> load shedding logic/1
  Compare To Constant/1 -> load shedding logic/2
  load shedding logic/1 -> trip/1
  V/1 -> frequency estimator (discrete)/1(v), RMS1/1
  frequency estimator (discrete)/1(w) -> Compare To Constant1/1, w/1, Compare To Constant2/1, Compare To Constant3/1, Compare To Constant4/1
  Compare To Constant1/1 -> Mux/1
  Compare To Constant2/1 -> Mux/2
  Compare To Constant3/1 -> Mux/3
  Compare To Constant4/1 -> Mux/4
  RMS1/1 -> Compare To Constant5/1, Vrms/1
  Compare To Constant5/1 -> load shedding logic/3
  Mux/1 -> load shedding logic/4

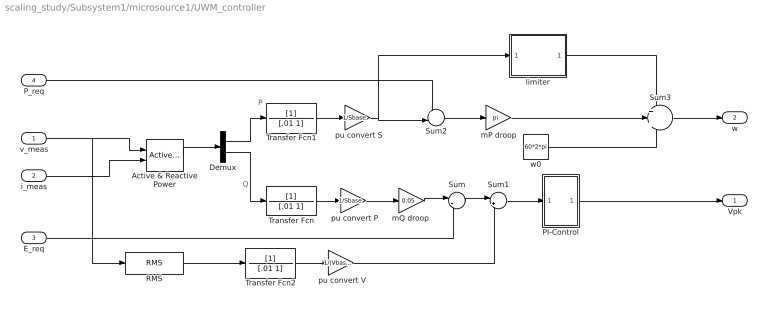
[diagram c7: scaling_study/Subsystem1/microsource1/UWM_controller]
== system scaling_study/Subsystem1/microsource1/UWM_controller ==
  note: P
  note: Q
  v_meas : Inport
  i_meas : Inport  Port=2
  E_req : Inport  Port=3
  P_req : Inport  Port=4
  " pu convert P" : Gain  Gain=1/Sbase  ParameterDataType=sfix(16)  ParameterScaling=2^0  OutDataType=sfix(16)  OutScaling=2^0
  " pu convert S" : Gain  Gain=1/Sbase  ParameterDataType=sfix(16)  ParameterScaling=2^0  OutDataType=sfix(16)  OutScaling=2^0
  " pu convert V" : Gain  Gain=1/(Vbase/sqrt(2))  ParameterDataType=sfix(16)  ParameterScaling=2^0  OutDataType=sfix(16)  OutScaling=2^0
  Active & Reactive Power : powerlib_extras/Measurements/Active & Reactive Power  DialogController=POWERSYS.PowerSysDialog  SystemSampleTime=-1  f1=60
  Demux : Demux  Outputs=2
  PI-Control : Subsystem
  RMS : powerlib_extras/Measurements/RMS  DialogController=POWERSYS.PowerSysDialog  SystemSampleTime=-1  f1=60
  Sum : Sum  Inputs=|-+  OutDataType=sfix(16)  OutScaling=2^0
  Sum1 : Sum  Inputs=|+-  OutDataType=sfix(16)  OutScaling=2^0
  Sum2 : Sum  Inputs=+-|  OutDataType=sfix(16)  OutScaling=2^0
  Sum3 : Sum  Inputs=+++  OutDataType=sfix(16)  OutScaling=2^0
  Transfer Fcn : TransferFcn  Denominator=[.01 1]
  Transfer Fcn1 : TransferFcn  Denominator=[.01 1]
  Transfer Fcn2 : TransferFcn  Denominator=[.01 1]
  limiter : Subsystem
  mP droop : Gain  Gain=pi  ParameterDataType=sfix(16)  ParameterScaling=2^0  OutDataType=sfix(16)  OutScaling=2^0
  "mQ droop " : Gain  Gain=0.05  ParameterDataType=sfix(16)  ParameterScaling=2^0  OutDataType=sfix(16)  OutScaling=2^0
  w0 : Constant  Value=60*2*pi  OutDataType=fixdt(1, 16)  OutScaling=2^0
  Vpk : Outport
  w : Outport  Port=2
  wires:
  Transfer Fcn2/1 -> " pu convert V"/1
  Transfer Fcn/1 -> " pu convert P"/1
  " pu convert P"/1 -> "mQ droop "/1
  Transfer Fcn1/1 -> " pu convert S"/1
  " pu convert S"/1 -> limiter/1(In1), Sum2/2
  i_meas/1 -> Active & Reactive Power/2
  P_req/1 -> Sum2/1
  mP droop/1 -> Sum3/2
  limiter/1(Out1) -> Sum3/1
  w0/1 -> Sum3/3
  Sum2/1 -> mP droop/1
  Sum1/1 -> PI-Control/1(In1)
  Sum/1 -> Sum1/1
  "mQ droop "/1 -> Sum/1
  Demux/2 -> Transfer Fcn/1
  Demux/1 -> Transfer Fcn1/1
  Active & Reactive Power/1 -> Demux/1
  v_meas/1 -> RMS/1, Active & Reactive Power/1
  PI-Control/1(Out1) -> Vpk/1
  Sum3/1 -> w/1
  E_req/1 -> Sum/2
  " pu convert V"/1 -> Sum1/2
  RMS/1 -> Transfer Fcn2/1

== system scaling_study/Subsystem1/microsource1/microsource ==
  Vpk : Inport  OutDataType=fixdt(1, 16)  OutScaling=2^0
  w : Inport  Port=2  OutDataType=fixdt(1, 16)  OutScaling=2^0
  Integrator : Integrator
  Product : Product  OutDataType=sfix(16)  OutScaling=2^0
  phaseA : powerlib/Electrical Sources/Controlled Voltage Source  DialogController=POWERSYS.PowerSysDialog  SystemSampleTime=-1  Initialize=on  Source_Type=AC  Amplitude=0  Phase=0  Frequency=0  Measurements=None
  v_A : Fcn  Expr=cos(u)
  Va : PMIOPort  Tag=PMCPort  Port=1  Side=Right
  Neutral : PMIOPort  Tag=PMCPort  Port=2  Side=Right
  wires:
  Product/1 -> phaseA/1
  Vpk/1 -> Product/1
  w/1 -> Integrator/1
  Integrator/1 -> v_A/1
  v_A/1 -> Product/2
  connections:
  phaseA/RConn1 -- Va/RConn1
  phaseA/LConn1 -- Neutral/RConn1

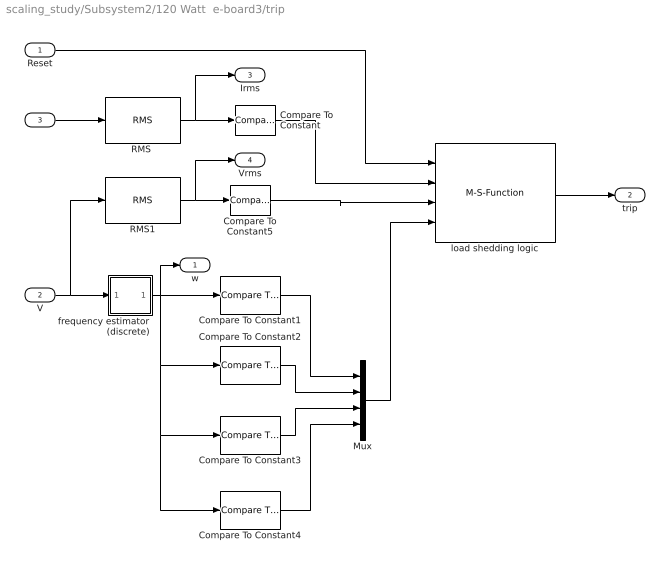
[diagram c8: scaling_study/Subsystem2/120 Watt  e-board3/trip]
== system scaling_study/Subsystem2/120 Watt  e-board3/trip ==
  Reset : Inport
  V : Inport  Port=2
  I : Inport  Port=3
  Compare To Constant : simulink/Logic and Bit Operations/Compare To Constant  SystemSampleTime=-1  relop=>=  const=100  LogicOutDataTypeMode=boolean
  Compare To Constant1 : simulink/Logic and Bit Operations/Compare To Constant  SystemSampleTime=-1  relop=<=  const=59.8  LogicOutDataTypeMode=boolean
  Compare To Constant2 : simulink/Logic and Bit Operations/Compare To Constant  SystemSampleTime=-1  relop=<=  const=59.5  LogicOutDataTypeMode=boolean
  Compare To Constant3 : simulink/Logic and Bit Operations/Compare To Constant  SystemSampleTime=-1  relop=>=  const=60.1  LogicOutDataTypeMode=boolean
  Compare To Constant4 : simulink/Logic and Bit Operations/Compare To Constant  SystemSampleTime=-1  relop=<=  const=58.6  LogicOutDataTypeMode=boolean
  Compare To Constant5 : simulink/Logic and Bit Operations/Compare To Constant  SystemSampleTime=-1  relop=<=  const=100  LogicOutDataTypeMode=boolean
  Mux : Mux
  "RMS " : powerlib_extras/Measurements/RMS  DialogController=POWERSYS.PowerSysDialog  SystemSampleTime=-1  f1=60
  RMS1 : powerlib_extras/Measurements/RMS  DialogController=POWERSYS.PowerSysDialog  SystemSampleTime=-1  f1=60
  frequency estimator (discrete) : Subsystem  mask{dt=0.010}
      mask prompts: dt "sample time"
  load shedding logic : M-S-Function  FunctionName=load_shedding_logic  Parameters=p
  w : Outport  OutDataType=fixdt(1, 16)  OutScaling=2^0
  trip : Outport  Port=2  DataType=double  OutDataTypeStr=double
  Irms : Outport  Port=3  OutDataType=fixdt(1, 16)  OutScaling=2^0
  Vrms : Outport  Port=4  OutDataType=fixdt(1, 16)  OutScaling=2^0
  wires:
  "RMS "/1 -> Compare To Constant/1, Irms/1
  I/1 -> "RMS "/1
  Reset/1 -> load shedding logic/1
  Compare To Constant/1 -> load shedding logic/2
  load shedding logic/1 -> trip/1
  V/1 -> frequency estimator (discrete)/1(v), RMS1/1
  frequency estimator (discrete)/1(w) -> Compare To Constant1/1, w/1, Compare To Constant2/1, Compare To Constant3/1, Compare To Constant4/1
  Compare To Constant1/1 -> Mux/1
  Compare To Constant2/1 -> Mux/2
  Compare To Constant3/1 -> Mux/3
  Compare To Constant4/1 -> Mux/4
  RMS1/1 -> Compare To Constant5/1, Vrms/1
  Compare To Constant5/1 -> load shedding logic/3
  Mux/1 -> load shedding logic/4

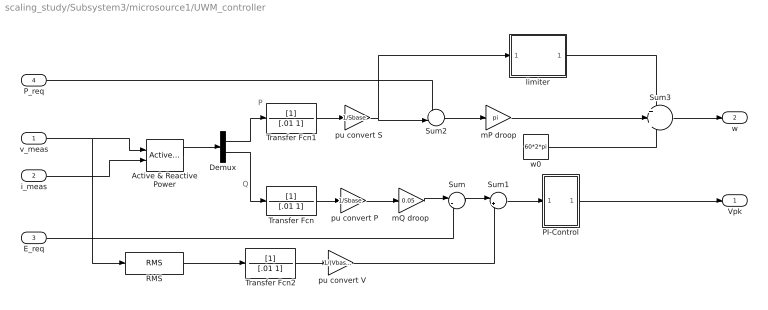
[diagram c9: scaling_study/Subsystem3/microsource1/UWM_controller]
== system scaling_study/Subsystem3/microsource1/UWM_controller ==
  note: P
  note: Q
  v_meas : Inport
  i_meas : Inport  Port=2
  E_req : Inport  Port=3
  P_req : Inport  Port=4
  " pu convert P" : Gain  Gain=1/Sbase  ParameterDataType=sfix(16)  ParameterScaling=2^0  OutDataType=sfix(16)  OutScaling=2^0
  " pu convert S" : Gain  Gain=1/Sbase  ParameterDataType=sfix(16)  ParameterScaling=2^0  OutDataType=sfix(16)  OutScaling=2^0
  " pu convert V" : Gain  Gain=1/(Vbase/sqrt(2))  ParameterDataType=sfix(16)  ParameterScaling=2^0  OutDataType=sfix(16)  OutScaling=2^0
  Active & Reactive Power : powerlib_extras/Measurements/Active & Reactive Power  DialogController=POWERSYS.PowerSysDialog  SystemSampleTime=-1  f1=60
  Demux : Demux  Outputs=2
  PI-Control : Subsystem
  RMS : powerlib_extras/Measurements/RMS  DialogController=POWERSYS.PowerSysDialog  SystemSampleTime=-1  f1=60
  Sum : Sum  Inputs=|-+  OutDataType=sfix(16)  OutScaling=2^0
  Sum1 : Sum  Inputs=|+-  OutDataType=sfix(16)  OutScaling=2^0
  Sum2 : Sum  Inputs=+-|  OutDataType=sfix(16)  OutScaling=2^0
  Sum3 : Sum  Inputs=+++  OutDataType=sfix(16)  OutScaling=2^0
  Transfer Fcn : TransferFcn  Denominator=[.01 1]
  Transfer Fcn1 : TransferFcn  Denominator=[.01 1]
  Transfer Fcn2 : TransferFcn  Denominator=[.01 1]
  limiter : Subsystem
  mP droop : Gain  Gain=pi  ParameterDataType=sfix(16)  ParameterScaling=2^0  OutDataType=sfix(16)  OutScaling=2^0
  "mQ droop " : Gain  Gain=0.05  ParameterDataType=sfix(16)  ParameterScaling=2^0  OutDataType=sfix(16)  OutScaling=2^0
  w0 : Constant  Value=60*2*pi  OutDataType=fixdt(1, 16)  OutScaling=2^0
  Vpk : Outport
  w : Outport  Port=2
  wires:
  Transfer Fcn2/1 -> " pu convert V"/1
  Transfer Fcn/1 -> " pu convert P"/1
  " pu convert P"/1 -> "mQ droop "/1
  Transfer Fcn1/1 -> " pu convert S"/1
  " pu convert S"/1 -> limiter/1(In1), Sum2/2
  i_meas/1 -> Active & Reactive Power/2
  P_req/1 -> Sum2/1
  mP droop/1 -> Sum3/2
  limiter/1(Out1) -> Sum3/1
  w0/1 -> Sum3/3
  Sum2/1 -> mP droop/1
  Sum1/1 -> PI-Control/1(In1)
  Sum/1 -> Sum1/1
  "mQ droop "/1 -> Sum/1
  Demux/2 -> Transfer Fcn/1
  Demux/1 -> Transfer Fcn1/1
  Active & Reactive Power/1 -> Demux/1
  v_meas/1 -> RMS/1, Active & Reactive Power/1
  PI-Control/1(Out1) -> Vpk/1
  Sum3/1 -> w/1
  E_req/1 -> Sum/2
  " pu convert V"/1 -> Sum1/2
  RMS/1 -> Transfer Fcn2/1

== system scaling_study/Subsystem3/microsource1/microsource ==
  Vpk : Inport  OutDataType=fixdt(1, 16)  OutScaling=2^0
  w : Inport  Port=2  OutDataType=fixdt(1, 16)  OutScaling=2^0
  Integrator : Integrator
  Product : Product  OutDataType=sfix(16)  OutScaling=2^0
  phaseA : powerlib/Electrical Sources/Controlled Voltage Source  DialogController=POWERSYS.PowerSysDialog  SystemSampleTime=-1  Initialize=on  Source_Type=AC  Amplitude=0  Phase=0  Frequency=0  Measurements=None
  v_A : Fcn  Expr=cos(u)
  Va : PMIOPort  Tag=PMCPort  Port=1  Side=Right
  Neutral : PMIOPort  Tag=PMCPort  Port=2  Side=Right
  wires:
  Product/1 -> phaseA/1
  Vpk/1 -> Product/1
  w/1 -> Integrator/1
  Integrator/1 -> v_A/1
  v_A/1 -> Product/2
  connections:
  phaseA/RConn1 -- Va/RConn1
  phaseA/LConn1 -- Neutral/RConn1

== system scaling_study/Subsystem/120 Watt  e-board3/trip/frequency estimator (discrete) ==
  v : Inport
  Constant : Constant  Value=60  OutDataType=fixdt(1, 16)  OutScaling=2^0
  Fcn : Fcn  Expr=sin(2*pi*u[1])
  Filter Quantized : Subsystem  Tag=BlockMethodSubSystem
  Gain : Gain  Gain=1/150  ParameterDataType=fixdt(1, 16)  ParameterScaling=2^0  OutDataType=fixdt(1, 16)  OutScaling=2^0  SampleTime=dt
  Product : Product  OutDataType=fixdt(1, 16)  OutScaling=2^0
  Scope : Scope
  Sum : Sum  Inputs=|++  OutDataType=fixdt(1, 16)  OutScaling=2^0
  modulo discrete integrator : Subsystem  mask{dt=dt}
      mask prompts: dt "sample time"
  w : Outport  OutDataType=fixdt(1, 16)  OutScaling=2^0
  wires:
  Fcn/1 -> Product/2
  Constant/1 -> Sum/2
  modulo discrete integrator/1(Out1) -> Fcn/1
  Sum/1 -> modulo discrete integrator/1(In1), w/1
  Product/1 -> Filter Quantized/1(In)
  Filter Quantized/1(Out) -> Scope/1, Sum/1
  v/1 -> Gain/1
  Gain/1 -> Product/1

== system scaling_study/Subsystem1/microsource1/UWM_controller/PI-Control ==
  In1 : Inport
  Gain : Gain  Gain=.01  ParameterDataType=sfix(16)  ParameterScaling=2^0  OutDataType=sfix(16)  OutScaling=2^0
  Gain1 : Gain  Gain=5  ParameterDataType=sfix(16)  ParameterScaling=2^0  OutDataType=sfix(16)  OutScaling=2^0
  Gain2 : Gain  Gain=750  ParameterDataType=sfix(16)  ParameterScaling=2^0  OutDataType=sfix(16)  OutScaling=2^0
  Integrator1 : Integrator  LimitOutput=on  UpperSaturationLimit=100  LowerSaturationLimit=-100  ZeroCross=off
  Sum4 : Sum  Inputs=|++  OutDataType=sfix(16)  OutScaling=2^0
  Out1 : Outport
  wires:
  Gain/1 -> Sum4/1
  Integrator1/1 -> Sum4/2
  In1/1 -> Gain1/1, Gain/1
  Gain1/1 -> Integrator1/1
  Sum4/1 -> Gain2/1
  Gain2/1 -> Out1/1

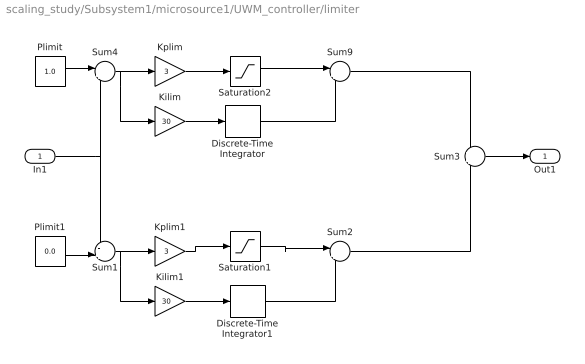
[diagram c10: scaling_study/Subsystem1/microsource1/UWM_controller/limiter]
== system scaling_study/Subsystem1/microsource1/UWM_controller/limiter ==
  In1 : Inport
  Discrete-Time Integrator : DiscreteIntegrator  OutDataType=fixdt(1, 16)  OutScaling=2^0  LimitOutput=on  UpperSaturationLimit=0  LowerSaturationLimit=-pi  ICPrevOutput=DiscIntNeverNeededParam  ICPrevScaledInput=DiscIntNeverNeededParam
  Discrete-Time Integrator1 : DiscreteIntegrator  OutDataType=fixdt(1, 16)  OutScaling=2^0  LimitOutput=on  UpperSaturationLimit=pi  LowerSaturationLimit=0  ICPrevOutput=DiscIntNeverNeededParam  ICPrevScaledInput=DiscIntNeverNeededParam
  Kilim : Gain  Gain=30  ParameterDataType=sfix(16)  ParameterScaling=2^0  OutDataType=sfix(16)  OutScaling=2^0
  Kilim1 : Gain  Gain=30  ParameterDataType=sfix(16)  ParameterScaling=2^0  OutDataType=sfix(16)  OutScaling=2^0
  Kplim : Gain  Gain=3  ParameterDataType=sfix(16)  ParameterScaling=2^0  OutDataType=sfix(16)  OutScaling=2^0
  Kplim1 : Gain  Gain=3  ParameterDataType=sfix(16)  ParameterScaling=2^0  OutDataType=sfix(16)  OutScaling=2^0
  Plimit : Constant  Value=1.0  OutDataType=sfix(16)  OutScaling=2^0
  Plimit1 : Constant  Value=0.0  OutDataType=sfix(16)  OutScaling=2^0
  Saturation1 : Saturate  UpperLimit=pi  LowerLimit=0  OutDataType=fixdt(1, 16)  OutScaling=2^0
  Saturation2 : Saturate  UpperLimit=0  LowerLimit=-pi  OutDataType=fixdt(1, 16)  OutScaling=2^0
  Sum1 : Sum  Inputs=-+|  OutDataType=sfix(16)  OutScaling=2^0
  Sum2 : Sum  Inputs=|++  OutDataType=sfix(16)  OutScaling=2^0
  Sum3 : Sum  OutDataType=sfix(16)  OutScaling=2^0
  Sum4 : Sum  Inputs=|+-  OutDataType=sfix(16)  OutScaling=2^0
  Sum9 : Sum  Inputs=|++  OutDataType=sfix(16)  OutScaling=2^0
  Out1 : Outport
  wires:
  Sum3/1 -> Out1/1
  Plimit1/1 -> Sum1/2
  Discrete-Time Integrator1/1 -> Sum2/2
  Kilim1/1 -> Discrete-Time Integrator1/1
  Sum1/1 -> Kilim1/1, Kplim1/1
  In1/1 -> Sum1/1, Sum4/2
  Discrete-Time Integrator/1 -> Sum9/2
  Kilim/1 -> Discrete-Time Integrator/1
  Sum4/1 -> Kilim/1, Kplim/1
  Plimit/1 -> Sum4/1
  Kplim1/1 -> Saturation1/1
  Saturation1/1 -> Sum2/1
  Kplim/1 -> Saturation2/1
  Saturation2/1 -> Sum9/1
  Sum9/1 -> Sum3/1
  Sum2/1 -> Sum3/2

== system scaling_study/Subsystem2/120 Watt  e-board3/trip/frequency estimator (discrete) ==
  v : Inport
  Constant : Constant  Value=60  OutDataType=fixdt(1, 16)  OutScaling=2^0
  Fcn : Fcn  Expr=sin(2*pi*u[1])
  Filter Quantized : Subsystem  Tag=BlockMethodSubSystem
  Gain : Gain  Gain=1/150  ParameterDataType=fixdt(1, 16)  ParameterScaling=2^0  OutDataType=fixdt(1, 16)  OutScaling=2^0  SampleTime=dt
  Product : Product  OutDataType=fixdt(1, 16)  OutScaling=2^0
  Scope : Scope
  Sum : Sum  Inputs=|++  OutDataType=fixdt(1, 16)  OutScaling=2^0
  modulo discrete integrator : Subsystem  mask{dt=dt}
      mask prompts: dt "sample time"
  w : Outport  OutDataType=fixdt(1, 16)  OutScaling=2^0
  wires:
  Fcn/1 -> Product/2
  Constant/1 -> Sum/2
  modulo discrete integrator/1(Out1) -> Fcn/1
  Sum/1 -> modulo discrete integrator/1(In1), w/1
  Product/1 -> Filter Quantized/1(In)
  Filter Quantized/1(Out) -> Scope/1, Sum/1
  v/1 -> Gain/1
  Gain/1 -> Product/1

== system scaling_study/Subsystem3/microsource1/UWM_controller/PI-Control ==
  In1 : Inport
  Gain : Gain  Gain=.01  ParameterDataType=sfix(16)  ParameterScaling=2^0  OutDataType=sfix(16)  OutScaling=2^0
  Gain1 : Gain  Gain=5  ParameterDataType=sfix(16)  ParameterScaling=2^0  OutDataType=sfix(16)  OutScaling=2^0
  Gain2 : Gain  Gain=750  ParameterDataType=sfix(16)  ParameterScaling=2^0  OutDataType=sfix(16)  OutScaling=2^0
  Integrator1 : Integrator  LimitOutput=on  UpperSaturationLimit=100  LowerSaturationLimit=-100  ZeroCross=off
  Sum4 : Sum  Inputs=|++  OutDataType=sfix(16)  OutScaling=2^0
  Out1 : Outport
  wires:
  Gain/1 -> Sum4/1
  Integrator1/1 -> Sum4/2
  In1/1 -> Gain1/1, Gain/1
  Gain1/1 -> Integrator1/1
  Sum4/1 -> Gain2/1
  Gain2/1 -> Out1/1

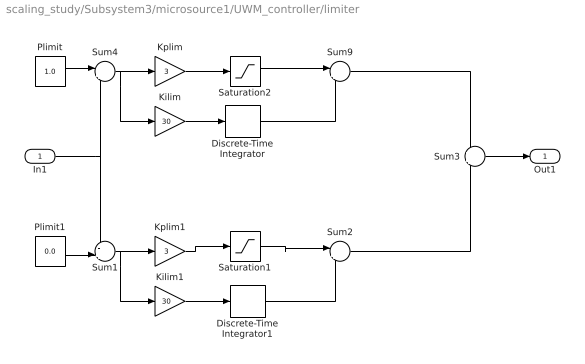
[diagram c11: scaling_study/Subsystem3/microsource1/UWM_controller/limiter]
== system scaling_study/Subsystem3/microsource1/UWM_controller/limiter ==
  In1 : Inport
  Discrete-Time Integrator : DiscreteIntegrator  OutDataType=fixdt(1, 16)  OutScaling=2^0  LimitOutput=on  UpperSaturationLimit=0  LowerSaturationLimit=-pi  ICPrevOutput=DiscIntNeverNeededParam  ICPrevScaledInput=DiscIntNeverNeededParam
  Discrete-Time Integrator1 : DiscreteIntegrator  OutDataType=fixdt(1, 16)  OutScaling=2^0  LimitOutput=on  UpperSaturationLimit=pi  LowerSaturationLimit=0  ICPrevOutput=DiscIntNeverNeededParam  ICPrevScaledInput=DiscIntNeverNeededParam
  Kilim : Gain  Gain=30  ParameterDataType=sfix(16)  ParameterScaling=2^0  OutDataType=sfix(16)  OutScaling=2^0
  Kilim1 : Gain  Gain=30  ParameterDataType=sfix(16)  ParameterScaling=2^0  OutDataType=sfix(16)  OutScaling=2^0
  Kplim : Gain  Gain=3  ParameterDataType=sfix(16)  ParameterScaling=2^0  OutDataType=sfix(16)  OutScaling=2^0
  Kplim1 : Gain  Gain=3  ParameterDataType=sfix(16)  ParameterScaling=2^0  OutDataType=sfix(16)  OutScaling=2^0
  Plimit : Constant  Value=1.0  OutDataType=sfix(16)  OutScaling=2^0
  Plimit1 : Constant  Value=0.0  OutDataType=sfix(16)  OutScaling=2^0
  Saturation1 : Saturate  UpperLimit=pi  LowerLimit=0  OutDataType=fixdt(1, 16)  OutScaling=2^0
  Saturation2 : Saturate  UpperLimit=0  LowerLimit=-pi  OutDataType=fixdt(1, 16)  OutScaling=2^0
  Sum1 : Sum  Inputs=-+|  OutDataType=sfix(16)  OutScaling=2^0
  Sum2 : Sum  Inputs=|++  OutDataType=sfix(16)  OutScaling=2^0
  Sum3 : Sum  OutDataType=sfix(16)  OutScaling=2^0
  Sum4 : Sum  Inputs=|+-  OutDataType=sfix(16)  OutScaling=2^0
  Sum9 : Sum  Inputs=|++  OutDataType=sfix(16)  OutScaling=2^0
  Out1 : Outport
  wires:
  Sum3/1 -> Out1/1
  Plimit1/1 -> Sum1/2
  Discrete-Time Integrator1/1 -> Sum2/2
  Kilim1/1 -> Discrete-Time Integrator1/1
  Sum1/1 -> Kilim1/1, Kplim1/1
  In1/1 -> Sum1/1, Sum4/2
  Discrete-Time Integrator/1 -> Sum9/2
  Kilim/1 -> Discrete-Time Integrator/1
  Sum4/1 -> Kilim/1, Kplim/1
  Plimit/1 -> Sum4/1
  Kplim1/1 -> Saturation1/1
  Saturation1/1 -> Sum2/1
  Kplim/1 -> Saturation2/1
  Saturation2/1 -> Sum9/1
  Sum9/1 -> Sum3/1
  Sum2/1 -> Sum3/2
